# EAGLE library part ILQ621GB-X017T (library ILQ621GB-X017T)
Transistor Output Optocouplers Phototransistor Out Quad CTR > 100% Source: Datasheet
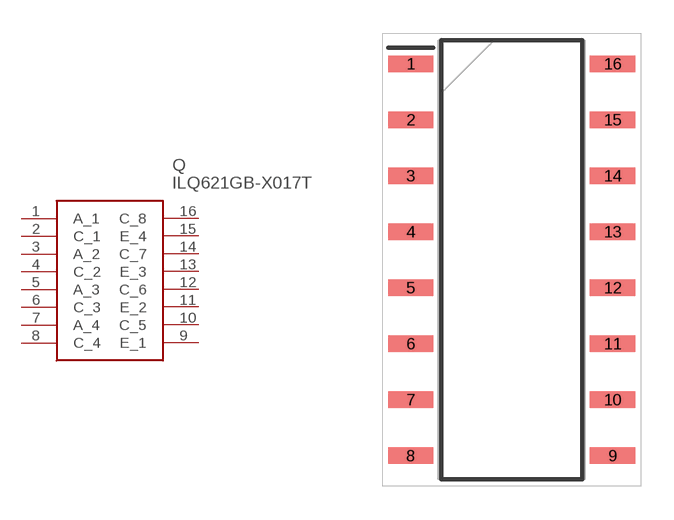
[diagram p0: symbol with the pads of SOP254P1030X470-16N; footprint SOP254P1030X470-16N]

Designator prefix Q

## ILQ621GB-X017T (Description: Transistor Output Optocouplers Phototransistor Out Quad CTR > 100%; Height: 4.7mm; Manufacturer_Name: Vishay; Manufacturer_Part_Number: ILQ621GB-X017T; Mouser_Part_Number: 782-ILQ621GB-X017T; Mouser_Price-Stock: https://www.mouser.co.uk/ProductDetail/Vishay-Semiconductors/ILQ621GB-X017T?qs=%2Fjqivxn91cep6dKZN8S1JQ%3D%3D)  [SOP254P1030X470-16N]
1  A_1
2  C_1
3  A_2
4  C_2
5  A_3
6  C_3
7  A_4
8  C_4
9  E_1
10  C_5
11  E_2
12  C_6
13  E_3
14  C_7
15  E_4
16  C_8

## Footprint SOP254P1030X470-16N (pad centres in mm)
ILQ621GB-X017T
smd 2.05 x 0.75: 1 -4.575,8.89; 2 -4.575,6.35; 3 -4.575,3.81; 4 -4.575,1.27; 5 -4.575,-1.27; 6 -4.575,-3.81; 7 -4.575,-6.35; 8 -4.575,-8.89; 9 4.575,-8.89; 10 4.575,-6.35; 11 4.575,-3.81; 12 4.575,-1.27; 13 4.575,1.27; 14 4.575,3.81; 15 4.575,6.35; 16 4.575,8.89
